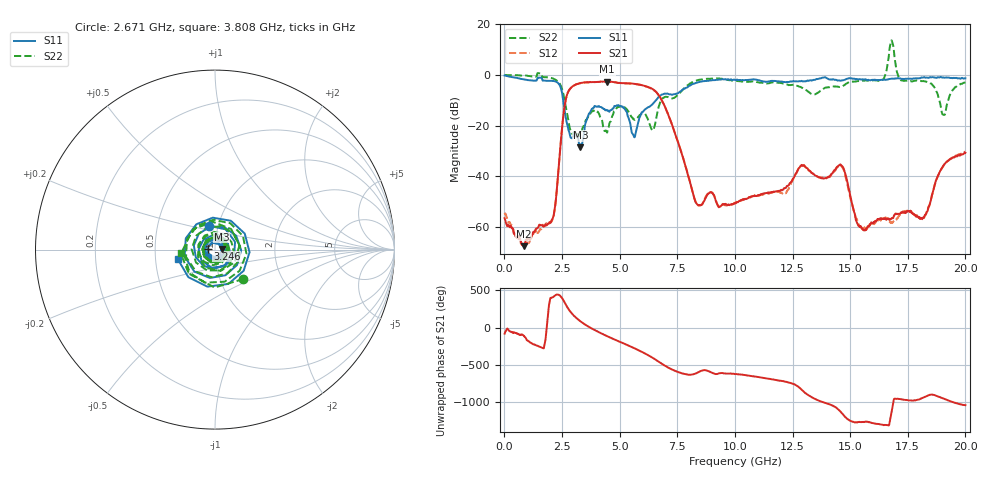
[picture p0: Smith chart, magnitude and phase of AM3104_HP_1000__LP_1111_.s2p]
!Created with skrf (http://scikit-rf.org).
# Hz S RI R 50.0
!freq ReS11 ImS11 ReS21 ImS21 ReS12 ImS12 ReS22 ImS22
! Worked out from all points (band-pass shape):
!   1601 points, 10 MHz to 20 GHz, reference 50 ohm
!   highest |S21| = -2.62 dB at 4.458 GHz (marker M1); lowest = -67.7 dB at 834.6 MHz (marker M2)
!   |S21| within 3 dB of the highest: 2.837 GHz to 6.434 GHz (3.597 GHz wide, 77.6 % of centre)
!   lowest |S11| = -28.6 dB at 3.296 GHz (marker M3), VSWR 1.08, Z = 53.8 + j0.315 ohm
!   |S11| at or under -10 dB: 2.548 GHz to 6.576 GHz (4.028 GHz wide, 88.3 % of centre)
!   |S22| runs from -24.4 to 13.6 dB; largest |S21 - S12| = 0.083
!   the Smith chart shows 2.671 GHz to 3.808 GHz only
!   S11 on the Smith chart (normalised r, x): 2.671 GHz: 0.91, +0.24; 3.246 GHz: 0.92, +0.01; 3.808 GHz: 0.65, -0.07
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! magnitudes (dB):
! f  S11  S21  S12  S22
! 10 MHz  -0.2  -56.6  -54.5  -0.1
! 834.6 MHz  -1.8  -67.7  -66.9  -0.2
! 2.096 GHz  -2.4  -56.7  -56.9  -1.4
! 2.671 GHz  -17.3  -9.4  -9.4  -12.8
! 3.246 GHz  -27.5  -3.3  -3.4  -23.7
! 3.296 GHz  -28.6  -3.2  -3.3  -23.2
! 3.346 GHz  -27.3  -3.1  -3.2  -22.6
! 3.808 GHz  -13.4  -2.8  -2.8  -14.3
! 4.458 GHz  -13.9  -2.6  -2.6  -22.8
! 4.97 GHz  -12.1  -3.1  -3.2  -12.6
! 5.62 GHz  -24.2  -3.5  -3.5  -17.5
! 6.682 GHz  -8.8  -7.8  -7.8  -13.0
! 8.343 GHz  -3.1  -50.9  -50.7  -2.2
! 10.01 GHz  -2.0  -50.7  -50.5  -2.4
! 13.34 GHz  -2.2  -38.8  -38.8  -7.6
! 14.64 GHz  -2.2  -35.9  -36.2  -4.6
! 15.58 GHz  -1.8  -61.3  -60.6  -2.3
! 16.4 GHz  -2.0  -56.9  -56.7  -1.9
! 16.68 GHz  -1.7  -57.0  -57.7  7.3
! 18.19 GHz  -1.0  -56.5  -56.2  -2.4
! 19.05 GHz  -1.0  -35.8  -35.8  -15.7
! 20 GHz  -1.3  -30.8  -30.4  -3.0
